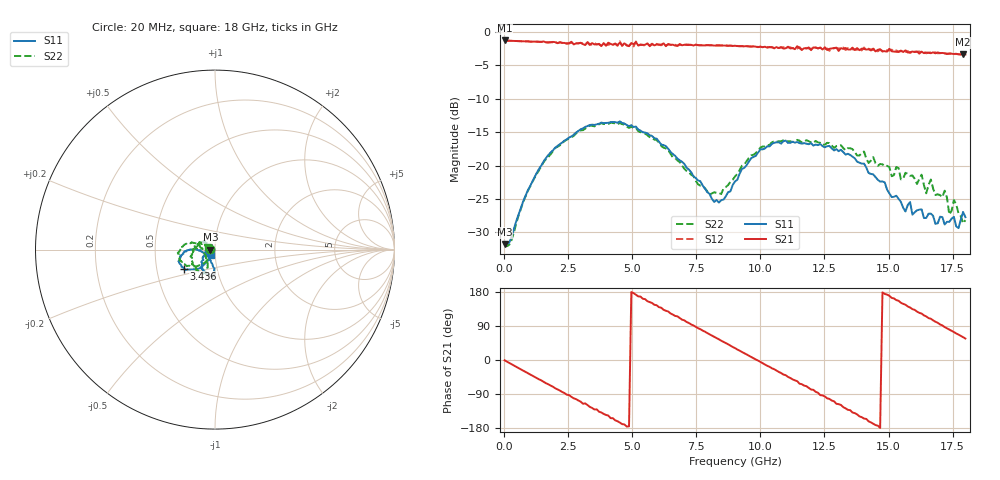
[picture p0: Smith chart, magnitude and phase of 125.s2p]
!Agilent Technologies,N5230A,US43500223,A.07.50.48
!Agilent N5230A: A.07.50.48
!Date: Sunday, January 17, 2016 20:56:44
!Correction: S11(Full 2 Port(1,2))
!S21(Full 2 Port(1,2))
!S12(Full 2 Port(1,2))
!S22(Full 2 Port(1,2))
!S2P File: Measurements: S11, S21, S12, S22:
# Hz S  dB  R 50
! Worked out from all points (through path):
!   201 points, 20 MHz to 18 GHz, reference 50 ohm
!   highest |S21| = -1.25 dB at 20 MHz (marker M1); lowest = -3.4 dB at 17.91 GHz (marker M2)
!   group delay of S21, straight-line fit = 102 ps
!   lowest |S11| = -31.8 dB at 20 MHz (marker M3), VSWR 1.05, Z = 47.5 + j0.0502 ohm
!   |S11| at or under -10 dB: start of sweep to end of sweep
!   |S22| runs from -32.1 to -13.6 dB; largest |S21 - S12| = 0.039
!   S11 on the Smith chart (normalised r, x): 20 MHz: 0.95, +0.00; 3.436 GHz: 0.69, -0.16; 18 GHz: 0.95, -0.06
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2e7  -31.81 178.8  -1.25 -0.8  -1.27 -0.9  -31.75 178.2
1.5483e9  -19.34 -126.4  -1.40 -57.8  -1.42 -57.8  -19.45 -129.6
2.6271e9  -15.63 -138.1  -1.45 -97.3  -1.58 -96.5  -15.76 -145.0
3.0766e9  -14.44 -144.5  -1.80 -115.5  -1.69 -114.2  -14.71 -152.0
3.4362e9  -13.88 -148.0  -1.66 -126.6  -1.84 -126.5  -14.04 -157.3
4.515e9  -13.38 -162.3  -1.57 -165.1  -1.38 -164.7  -13.63 -175.0
5.1443e9  -14.17 -170.1  -1.51 172.3  -1.41 173.3  -14.35 176.0
6.0433e9  -16.41 -178.6  -1.88 139.4  -1.90 138.6  -16.59 165.5
7.4817e9  -21.89 -174.8  -1.87 87.5  -1.92 87.3  -22.32 173.2
8.3807e9  -25.56 -141.3  -1.97 54.7  -2.01 54.5  -24.11 -148.9
9.01e9  -22.39 -105.9  -2.04 31.4  -2.11 31.5  -21.65 -120.2
1.02686e10  -17.11 -90.7  -2.34 -15.4  -2.22 -15.0  -16.99 -115.4
1.11676e10  -16.60 -98.9  -2.45 -47.4  -2.29 -48.3  -16.38 -127.1
1.20666e10  -17.01 -110.9  -2.30 -78.7  -2.50 -79.9  -16.61 -145.6
1.29656e10  -17.54 -118.4  -2.33 -115.5  -2.37 -112.6  -17.09 -163.0
1.35949e10  -18.66 -128.7  -2.33 -138.6  -2.57 -136.9  -17.55 -171.7
1.40444e10  -19.71 -137.4  -2.52 -154.5  -2.31 -153.7  -17.89 -179.3
1.50333e10  -24.17 -157.5  -2.50 169.3  -2.77 169.1  -20.23 164.6
1.63818e10  -27.86 -175.0  -3.16 117.7  -2.93 117.8  -22.93 147.2
1.77303e10  -29.38 -134.0  -3.34 67.1  -3.29 66.3  -27.17 178.3
1.79101e10  -26.96 -120.0  -3.36 60.1  -3.31 59.8  -28.66 157.9
1.8e10  -27.74 -127.3  -3.36 56.7  -3.37 56.3  -28.19 161.5
